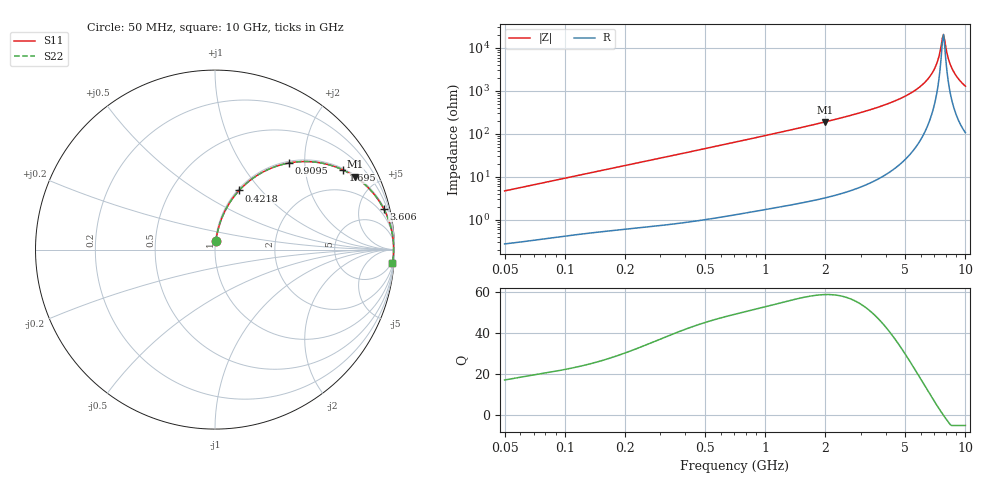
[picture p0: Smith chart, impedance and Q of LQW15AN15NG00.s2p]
!Murata Part Number: LQW15AN15NG00
!These Parameters are Measured in Series Mode Connection
!  o--[Z]--o
!Port1  Port2
!  o-------o
!Freq. Start=50[MHz] Stop=10[GHz], 401[Steps]
# Hz S RI R 50
!Freq.(Hz)	S 11(Real)	S 11(Imag)	S 21(Real)	S 21(Imag)	S 12(Real)	S 12(Imag)	S 22(Real)	S 22(Imag)
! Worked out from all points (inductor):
!   401 points, 50 MHz to 10 GHz, reference 50 ohm
!   read as one part in series: L = 15 nH near 51.34 MHz
!   highest Q = 58.6 at 1.987 GHz (marker M1), where L = 15.2 nH
!   self-resonance near 7.673 GHz
!   S11 on the Smith chart (normalised r, x): 50 MHz: 1.01, +0.09; 421.8 MHz: 1.02, +0.77; 909.5 MHz: 1.03, +1.66; 1.695 GHz: 1.06, +3.19; 3.606 GHz: 1.17, +8.18; 10 GHz: 3, -26
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5e7  0.00497 0.0469  0.995 -0.0469  0.995 -0.0469  0.00497 0.0469
1.214486e8  0.017 0.1101  0.983 -0.1101  0.983 -0.1101  0.017 0.1101
2.949953e8  0.0736 0.2478  0.9264 -0.2478  0.9264 -0.2478  0.0736 0.2478
4.218272e8  0.1346 0.3298  0.8654 -0.3298  0.8654 -0.3298  0.1346 0.3298
7.071068e8  0.2974 0.447  0.7026 -0.447  0.7026 -0.447  0.2974 0.447
9.094607e8  0.4105 0.4823  0.5895 -0.4823  0.5895 -0.4823  0.4105 0.4823
1.694942e9  0.7144 0.4431  0.2856 -0.4431  0.2856 -0.4431  0.7144 0.4431
1.717543e9  0.7202 0.4404  0.2798 -0.4404  0.2798 -0.4404  0.7202 0.4404
1.986945e9  0.7796 0.4061  0.2204 -0.4061  0.2204 -0.4061  0.7796 0.4061
3.606216e9  0.9394 0.2284  0.0606 -0.2284  0.0606 -0.2284  0.9394 0.2284
4.171863e9  0.9603 0.1834  0.0397 -0.1834  0.0397 -0.1834  0.9603 0.1834
5.437278e9  0.9847 0.1039  0.0153 -0.1039  0.0153 -0.1039  0.9847 0.1039
6.458996e9  0.9927 0.0536  0.00731 -0.0536  0.00731 -0.0536  0.9927 0.0536
7.086521e9  0.9947 0.0266  0.00527 -0.0266  0.00527 -0.0266  0.9947 0.0266
7.276762e9  0.995 0.0189  0.00498 -0.0189  0.00498 -0.0189  0.995 0.0189
7.571744e9  0.9952 0.00732  0.00478 -0.00732  0.00478 -0.00732  0.9952 0.00732
7.775012e9  0.9952 -0.000415  0.0048 0.000415  0.0048 0.000415  0.9952 -0.000415
7.878683e9  0.9951 -0.00429  0.00487 0.00429  0.00487 0.00429  0.9951 -0.00429
8.307378e9  0.9945 -0.0199  0.00545 0.0199  0.00545 0.0199  0.9945 -0.0199
8.644138e9  0.9937 -0.0316  0.00626 0.0316  0.00626 0.0316  0.9937 -0.0316
9.236013e9  0.9917 -0.0514  0.00833 0.0514  0.00833 0.0514  0.9917 -0.0514
1e10  0.9879 -0.0756  0.0121 0.0756  0.0121 0.0756  0.9879 -0.0756
